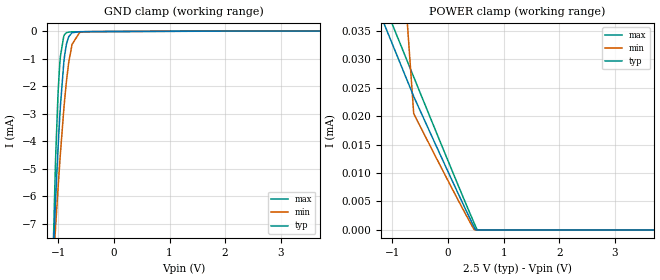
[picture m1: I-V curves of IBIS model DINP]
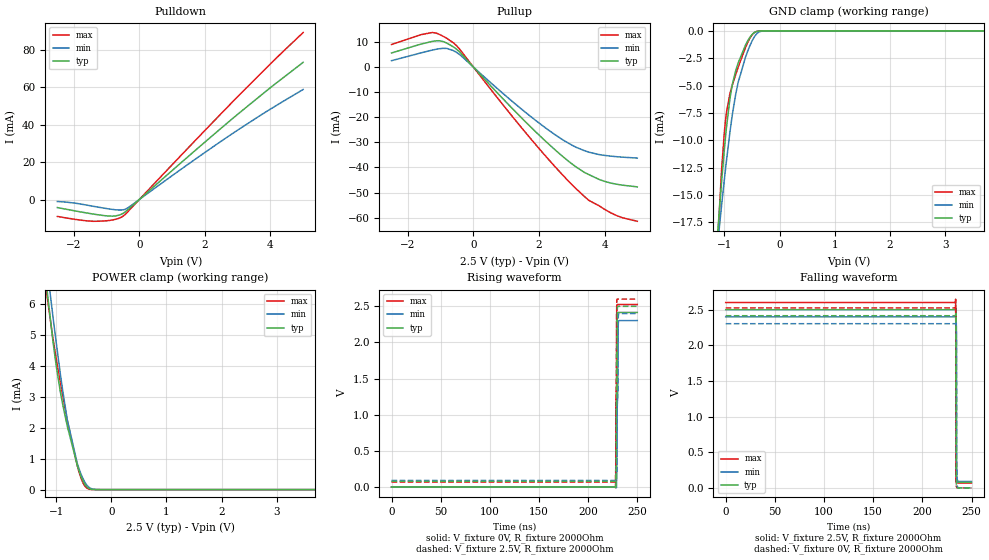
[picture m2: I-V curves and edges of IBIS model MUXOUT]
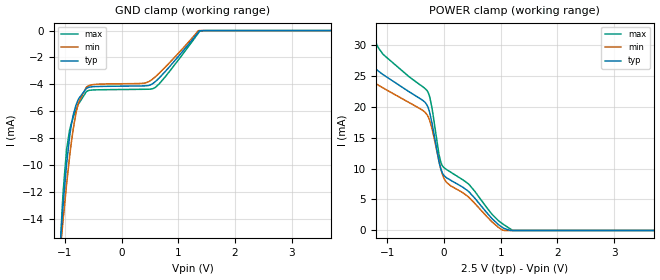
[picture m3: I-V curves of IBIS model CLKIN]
| Texas Instruments Incorporated
| Wideband Frequency Multiplier/Buffer/Divider
| Marketing part#   Voltage Range   Package-type   #pins/pkg drawing
| LMX1205RHA   2.4V - 2.6V   VQFN   40/ RHA
[IBIS Ver]   4.1
[File name]   lmx1205.ibs
[File Rev]   1.0
[Date]   18/12/2024
[Source]   Model built from spectre simulations at:
   Texas Instruments Incorporated.
   Analog-eLab, HPA
   12500 TI Blvd
   Dallas, TX -75243
   For Support e-mail: elab_ibis@list.ti.com
[Notes]   Revision History
   Rev 1.0: 18/12/2024
   | - Initial version of the model
   | - Model generated from simulations in TISPICE/SPECTRE
   | - C_comp although listed in numerical order of value are
   | obtained from varying PVT conditions. For PVT conditions for
   | each specific value refer the buffer description under
   | respective [Model]. IBIS model user is responsible for using
   | appropriate C_comp to simulate for Signal Integrity.
   | - Warnings regarding combined Non-monotonicity of various models have been
   | reviewed and considered minor and can be ignored.
[Disclaimer]  This model is designed as an aid for customers of Texas Instruments
 TI and its licensors and suppliers make no warranties, either expressed
 or implied, with respect to this  model, including the warranties of
 merchantability or fitness for a particular purpose.
 The model is provided solely on an "as is" basis. The entire risk as to
 its quality and performance is with the customer.
[Copyright] (C)Copyright 2024 Texas Instruments Incorporated.
   All rights reserved.
[Component]   LMX1205RHA
[Manufacturer]  Texas Instruments Incorporated
[Package]   | 40 QFN package
|   typ   min   max
R_pkg   0.342   0.082   0.685
L_pkg   0.157n   0.128n   0.174n
C_pkg   0.340p   0.293p   0.376p
[Pin]   signal_name   model_name   R_pin   L_pin   C_pin
1   MUXOUT   MUXOUT   0.191   0.157n   0.301p
2   SYSREFREQ_P   SYSREFREQ   0.081   0.136n   0.370p
3   SYSREFREQ_M   SYSREFREQ   0.115   0.136n   0.364p
4   VCC_CLKIN   POWER   0.118   0.128n   0.376p
5   GND   GND   0.116   0.136n   0.366p
6   CLKIN_P   CLKIN   0.089   0.139n   0.352p
7   CLKIN_M   CLKIN   0.098   0.138n   0.357p
8   SCK   DINP   0.155   0.149n   0.316p
9   SDI   DINP   0.116   0.156n   0.298p
10   CSB   DINP   0.166   0.160n   0.293p
11   SYSREFOUT0_M   SYSREFOUT   0.650   0.174n   0.339p
12   SYSREFOUT0_P   SYSREFOUT   0.652   0.166n   0.357p
13   GND   GND   0.657   0.160n   0.355p
14   CLKOUT0_M   CLKOUT   0.685   0.167n   0.331p
15   CLKOUT0_P   CLKOUT   0.648   0.133n   0.328p
16   VCC01   POWER   0.643   0.164n   0.340p
17   GND   GND   0.654   0.164n   0.337p
18   CLKOUT1_M   CLKOUT   0.650   0.163n   0.339p
19   CLKOUT1_P   CLKOUT   0.648   0.167n   0.349p
20   BIAS01   NC   0.656   0.164n   0.344p
21   SYSREFOUT1_M   SYSREFOUT   0.342   0.157n   0.336p
22   SYSREFOUT1_P   SYSREFOUT   0.330   0.145n   0.343p
23   LOGISYSREFOUT_M FPGAOUT   0.480   0.165n   0.302p
24   LOGISYSREFOUT_P FPGAOUT   0.486   0.166n   0.291p
25   VCC_LOGICLK   POWER   0.340   0.143n   0.346p
26   GND   GND   0.347   0.141n   0.358p
27   LOGICLKOUT_M   FPGAOUT   0.473   0.148n   0.312p
28   LOGICLKOUT_P   FPGAOUT   0.487   0.158n   0.310p
29   SYSREFOUT2_M   SYSREFOUT   0.365   0.151n   0.334p
30   SYSREFOUT2_P   SYSREFOUT   0.363   0.161n   0.332p
31   BIAS23   NC   0.656   0.164n   0.344p
32   CLKOUT2_M   CLKOUT   0.648   0.167n   0.349p
33   CLKOUT2_P   CLKOUT   0.650   0.163n   0.339p
34   GND   GND   0.654   0.164n   0.337p
35   VCC23   POWER   0.643   0.164n   0.340p
36   CLKOUT3_M   CLKOUT   0.648   0.133n   0.328p
37   CLKOUT3_P   CLKOUT   0.685   0.167n   0.331p
38   GND   GND   0.657   0.160n   0.355p
39   SYSREFOUT3_M   SYSREFOUT   0.652   0.166n   0.357p
40   SYSREFOUT3_P   SYSREFOUT   0.650   0.174n   0.339p
[Diff pin]  inv_pin  vdiff  tdelay_typ  tdelay_min  tdelay_max
  2   3   NA   NA   NA   NA
  6   7   NA   NA   NA   NA
 12   11   NA   0.0s   0.0s   0.0s
 15   14   NA   0.0s   0.0s   0.0s
 19   18   NA   0.0s   0.0s   0.0s
 22   21   NA   0.0s   0.0s   0.0s
 24   23   NA   0.0s   0.0s   0.0s
 28   27   NA   0.0s   0.0s   0.0s
 30   29   NA   0.0s   0.0s   0.0s
 33   32   NA   0.0s   0.0s   0.0s
 37   36   NA   0.0s   0.0s   0.0s
 40   39   NA   0.0s   0.0s   0.0s
| Models and submodels in the file (7): DINP (Input), MUXOUT (Output), CLKIN (Input), SYSREFREQ (Input), CLKOUT (Output), SYSREFOUT (Output), FPGAOUT (Output)
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|   Model DINP
[Model]   DINP
Model_type   Input
Vinl = 0.4
Vinh = 1.4
|   typ   min   max
C_comp   0.039pF   0.038pF   0.053pF
[Voltage Range]   2.5   2.4   2.6
[Temperature Range]   27   105   -40
[Power Clamp Reference]   2.5   2.4   2.6
[GND Clamp Reference]   0   0   0
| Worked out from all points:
|   GND clamp passes 1 mA (typ) near -0.89 V on its own axis
|   POWER clamp passes 1 mA (typ) near -1.77 V on its own axis
[GND Clamp]
|   Voltage   I(typ)   I(min)   I(max)
-2.5V     -98.77mA   -67mA      -178.3mA
-1.113V   -9.214mA   -9.271mA   -9.488mA
-1.052V   -6.289mA   -7.225mA   -4.881mA
-1.008V   -4.353mA   -5.784mA   -2.395mA
-977.5mV  -3.227mA   -4.879mA   -1.301mA
-962.5mV  -2.723mA   -4.446mA   -919.5uA
-902.5mV  -1.168mA   -2.872mA   -191.6uA
-850mV    -439uA     -1.752mA   -54.06uA
-812.5mV  -200.5uA   -1.133mA   -34.68uA
-752.5mV  -60.53uA   -480.4uA   -28.98uA
-572.5mV  -22.36uA   -31.33uA   -23.6uA
5V        0A         0A         0A
[POWER Clamp]
|   Voltage   I(typ)   I(min)   I(max)
-2.5V     12.91mA    14.05mA    11.79mA
-1.337V   40.69uA    120.2uA    44.17uA
-617.5mV  23.45uA    20.44uA    26.87uA
80mV      8.542uA    7.14uA     10.25uA
470mV     505.5nA    64.02nA    1.197uA
492.5mV   66.17nA    0A         693.7nA
522.5mV   0A         0A         29.53nA
537.5mV   0A         0A         0A
5V        0A         0A         0A
|   Model MUXOUT
[Model]   MUXOUT
Model_type   Output
Polarity   Non-Inverting
Vmeas = 1.25
Vref = 1.25
Cref = 2pF
Rref = 50
|   typ   min   max
C_comp   0.711pF   0.663pF   0.727pF
[Voltage Range]   2.5   2.4   2.6
[Temperature Range]   27   105   -40
[Pullup Reference]   2.5   2.4   2.6
[Pulldown Reference]   0   0   0
[Power Clamp Reference]   2.5   2.4   2.6
[GND Clamp Reference]   0   0   0
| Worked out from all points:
|   slope of the pulldown table from 0 to 0.375 V, typ, clamps not added: 64.4 ohm
|   slope of the pullup table from 0 to 0.375 V, typ, clamps not added: 70.4 ohm
|   GND clamp passes 1 mA (typ) near -0.59 V on its own axis
|   POWER clamp passes 1 mA (typ) near -0.65 V on its own axis
|   falling waveform, V_fixture 2.5V, R_fixture 2000Ohm: 20-80 % time 146ps typ, 178ps min, 91.2ps max; typ from 2.5 V to 0.078 V
|   rising waveform, V_fixture 0V, R_fixture 2000Ohm: 20-80 % time 889ps typ, 1.06ns min, 776ps max; typ from 0 V to 2.42 V
|   rising waveform, V_fixture 2.5V, R_fixture 2000Ohm: 20-80 % time 885ps typ, 1.06ns min, 774ps max; typ from 0.078 V to 2.5 V
|   falling waveform, V_fixture 0V, R_fixture 2000Ohm: 20-80 % time 147ps typ, 183ps min, 90.9ps max; typ from 2.42 V to 0 V
[Pulldown]
|   Voltage   I(typ)   I(min)   I(max)
-2.5V     -4.294mA   -1.047mA   -9.026mA
-1.99V    -5.977mA   -1.854mA   -10.51mA
-1.397V   -7.78mA    -3.629mA   -11.63mA
-820mV    -8.886mA   -5.277mA   -10.93mA
-617.5mV  -8.332mA   -5.605mA   -9.99mA
-490mV    -7.341mA   -5.484mA   -8.816mA
-317.5mV  -4.944mA   -4.066mA   -5.915mA
1.377V    21.24mA    17.46mA    25.5mA
2.788V    42.42mA    34.61mA    51.15mA
3.89V     58.23mA    47.13mA    70.54mA
5V        73.34mA    58.83mA    89.27mA
[GND Clamp]
|   Voltage   I(typ)   I(min)   I(max)
-2.5V     -131.9mA   -98.62mA   -211.9mA
-1.113V   -17.77mA   -18.95mA   -18.24mA
-1.052V   -13.84mA   -15.98mA   -12.75mA
-1V       -10.74mA   -13.51mA   -9.165mA
-962.5mV  -8.799mA   -11.83mA   -7.439mA
-902.5mV  -6.288mA   -9.349mA   -5.784mA
-850mV    -4.746mA   -7.442mA   -4.834mA
-752.5mV  -2.953mA   -4.728mA   -3.346mA
-565mV    -802.8uA   -1.689mA   -930.7uA
-437.5mV  -108.7uA   -399.2uA   -101.2uA
-197.5mV  -105.7nA   -1.103uA   -28.32nA
5V        0A         0A         0A
[Pullup]
|   Voltage   I(typ)   I(min)   I(max)
-2.5V     5.635mA    2.559mA    9.001mA
-1.27V    10.21mA    6.739mA    13.76mA
-925mV    10.19mA    7.48mA     12.28mA
-617.5mV  8.109mA    6.62mA     9.731mA
-422.5mV  6.025mA    4.992mA    7.158mA
1.752V    -23.92mA   -19.74mA   -28.6mA
2.518V    -33.26mA   -27.17mA   -40.07mA
3.058V    -39.06mA   -31.45mA   -47.52mA
3.53V     -42.88mA   -33.92mA   -53.16mA
4.175V    -46.15mA   -35.45mA   -57.95mA
4.543V    -47.03mA   -35.88mA   -59.99mA
5V        -47.71mA   -36.24mA   -61.44mA
[POWER Clamp]
|   Voltage   I(typ)   I(min)   I(max)
-2.5V     43.46mA    42.28mA    45.12mA
-1.188V   6.81mA     7.526mA    6.555mA
-1.06V    4.836mA    5.632mA    4.922mA
-992.5mV  3.937mA    4.675mA    4.18mA
-925mV    3.18mA     3.765mA    3.476mA
-797.5mV  2.051mA    2.259mA    2.238mA
-617.5mV  795.4uA    852.2uA    780.1uA
-587.5mV  626uA      689.1uA    589.1uA
-505mV    252uA      325.2uA    192.1uA
-430mV    65.99uA    117.4uA    34.14uA
-197.5mV  54.61nA    568nA      566.4pA
5V        0A         0A         0A
[Ramp]
R_load = 2000
|   typ   min   max
dV/dt_r   1.44932/8.88708e-10   1.38209/1.06338e-09   1.5153/7.76443e-10
dV/dt_f   1.45335/1.45865e-10   1.38614/1.78076e-10   1.51925/9.11995e-11
[Falling Waveform]
V_fixture = 2.5V
V_fixture_min = 2.4V
V_fixture_max = 2.6V
R_fixture = 2000Ohm
C_fixture = 0F
|   Time   V(typ)   V(min)   V(max)
0s        2.5V       2.4V       2.6V
233.8ns   2.515V     2.4V       2.648V
234ns     2.531V     2.408V     2.161V
234.1ns   2.376V     2.418V     495.6mV
234.2ns   2.327V     2.423V     150.6mV
234.3ns   1.463V     2.445V     109.5mV
234.5ns   167mV      2.277V     89.22mV
234.9ns   99.11mV    336.2mV    74.76mV
235.2ns   88.26mV    136.3mV    70.72mV
249.9ns   77.76mV    89.78mV    67.93mV
[Rising Waveform]
V_fixture = 0V
V_fixture_min = 0V
V_fixture_max = 0V
R_fixture = 2000Ohm
C_fixture = 0F
|   Time   V(typ)   V(min)   V(max)
0s        -6.212uV   -6.053uV   -6.38uV
227.8ns   38.53uV    5.753uV    -11.81mV
228.4ns   189.7mV    -13.72uV   1.266V
228.6ns   1.005V     -352.9uV   1.314V
228.9ns   1.225V     173.5mV    2.32V
229.1ns   1.282V     198.5mV    2.507V
229.6ns   2.371V     1.151V     2.525V
230ns     2.414V     1.282V     2.526V
230.7ns   2.416V     2.284V     2.526V
249.9ns   2.416V     2.303V     2.526V
[Rising Waveform]
V_fixture = 2.5V
V_fixture_min = 2.4V
V_fixture_max = 2.6V
R_fixture = 2000Ohm
C_fixture = 0F
|   Time   V(typ)   V(min)   V(max)
0s        77.76mV    89.78mV    67.93mV
227.8ns   77.81mV    89.79mV    55.91mV
228.4ns   260.8mV    89.77mV    1.307V
228.6ns   1.057V     89.43mV    1.357V
228.9ns   1.273V     258.7mV    2.397V
229.1ns   1.332V     280.9mV    2.582V
229.6ns   2.456V     1.208V     2.6V
230ns     2.498V     1.346V     2.6V
230.7ns   2.5V       2.381V     2.6V
249.9ns   2.5V       2.4V       2.6V
[Falling Waveform]
|Gnd
V_fixture = 0V
V_fixture_min = 0V
V_fixture_max = 0V
R_fixture = 2000Ohm
C_fixture = 0F
|   Time   V(typ)   V(min)   V(max)
0s        2.416V     2.303V     2.526V
233.8ns   2.43V      2.304V     2.565V
234ns     2.436V     2.311V     2.059V
234.1ns   2.282V     2.32V      391.2mV
234.2ns   2.221V     2.318V     76.21mV
234.3ns   1.276V     2.336V     38.92mV
234.5ns   79.09mV    2.166V     20.34mV
234.9ns   19.97mV    205.8mV    6.617mV
235.1ns   12.57mV    55.28mV    3.667mV
249.9ns   -6.492uV   -6.296uV   -6.657uV
|   Model CLKIN
[Model]   CLKIN
Model_type   Input
Vinl = 0.4
Vinh = 1.4
|   typ   min   max
C_comp   0.346pF   0.289pF   0.409pF
[Voltage Range]   2.5   2.4   2.6
[Temperature Range]   27   105   -40
[Power Clamp Reference]   2.5   2.4   2.6
[GND Clamp Reference]   0   0   0
[GND Clamp]
|   Voltage   I(typ)   I(min)   I(max)
-2.5V     -133.8mA   -105.7mA   -212.4mA
-1.15V    -20.19mA   -19.93mA   -22.83mA
-1.052V   -14.17mA   -15.11mA   -13.62mA
-1.03V    -12.92mA   -14.06mA   -11.98mA
-970mV    -9.965mA   -11.45mA   -8.86mA
-880mV    -6.881mA   -8.157mA   -6.827mA
-760mV    -5.097mA   -5.348mA   -5.47mA
-617.5mV  -4.291mA   -4.197mA   -4.528mA
417.5mV   -4.116mA   -3.902mA   -4.371mA
575mV     -3.873mA   -3.519mA   -4.285mA
1.355V    -135.5uA   -9.514uA   -187.9uA
5V        0A         0A         0A
[POWER Clamp]
|   Voltage   I(typ)   I(min)   I(max)
-2.5V     97.75mA    76.87mA    127.8mA
-1.893V   52.33mA    39.09mA    73.99mA
-1.6V     35.57mA    27.55mA    54.83mA
-1.472V   28.85mA    25.74mA    47.19mA
-1.225V   26.21mA    23.84mA    31.06mA
-1.075V   25.15mA    23mA       28.42mA
-280mV    19.81mA    18.35mA    22.26mA
-85mV     10.94mA    11.01mA    12.08mA
-25mV     9.202mA    8.972mA    10.38mA
440mV     6.225mA    5.322mA    7.422mA
1.032V    482.3uA    59.33uA    1.079mA
5V        0A         0A         0A
